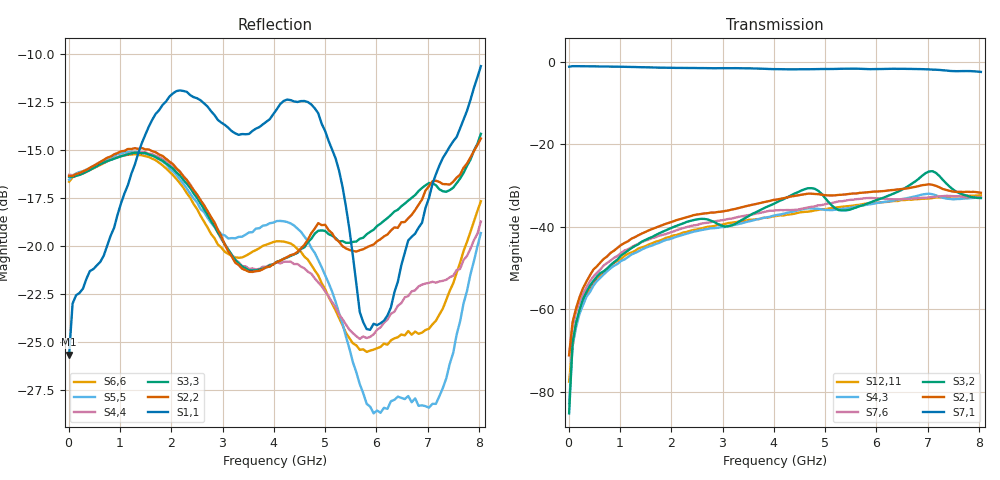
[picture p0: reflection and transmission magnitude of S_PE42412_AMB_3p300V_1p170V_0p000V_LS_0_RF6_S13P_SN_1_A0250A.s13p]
! Device ID: PE42412
! File Path: z:\PE42412\TE_GND_Post_Char_S-Param\All Parts\AMB\3p300\LS_0_RF6\PE42412_AMB_3p300V_1p170V_0p000V_LS_0_RF6_S13P_SN_1_A0250A.s13p
! Serial: 1
! Lot: A0250A
! Temp: AMB
! VDD: 3.300
! VSS: 0.000
! Control_Hi: 1.170
! Control_Lo: 0.000
! Logic State: LS_0_RF6
! Port 1:
! Port 2:
! Port 3:
! Port 4:
! Port 5:
! Port 6:
! Port 7:
! Port 8:
! Port 9:
! Port 10:
! Port 11:
! Port 12:
! Port 13:
! ThroughPath:1-7
! IDD: 0.0001070611
! ISS/IDD2: 5.72e-008
! IDMM3/IDD3: -1.926e-007
! Comment:
#  Hz  S  RI  R  50
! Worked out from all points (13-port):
!   120 points, 10 MHz to 8.037 GHz, reference 50 ohm
!   strongest paths, dB at 10 MHz, 2.034 GHz, 4.057 GHz, 6.08 GHz, 8.037 GHz:
!     S7,1: -1.1, -1.4, -1.7, -1.7, -2.4
!     S2,1: -71.1, -38.7, -33.4, -31.4, -31.7
!     S3,2: -85.2, -40.1, -34.0, -33.2, -33.0
!     S7,6: -71.1, -41.1, -36.0, -33.1, -32.8
!     S4,3: -82.8, -42.7, -37.1, -34.1, -32.9
!     S12,11: -77.5, -42.1, -37.3, -34.0, -32.3
!   lowest |S11| = -25.7 dB at 10 MHz (marker M1), VSWR 1.11, Z = 55.1 - j2.05 ohm
!   |S11| at or under -10 dB: start of sweep to end of sweep
